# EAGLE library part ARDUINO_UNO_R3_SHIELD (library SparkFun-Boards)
Arduino R3 Shield Footprint Shield form compatible with the Arduino Uno R3. SparkFun Products: MG2639 Cellular Shield MIDI Shield R3 Stackable Headers Kit
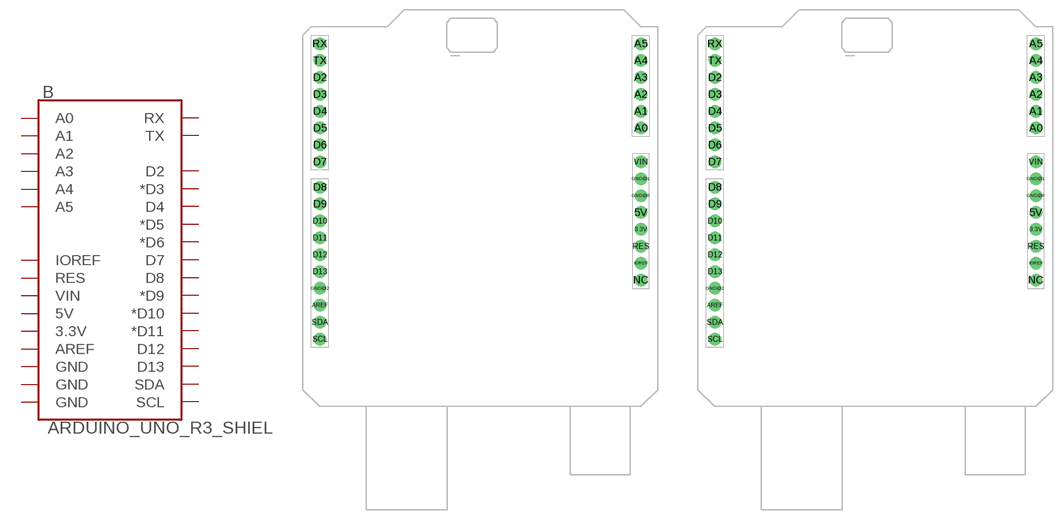
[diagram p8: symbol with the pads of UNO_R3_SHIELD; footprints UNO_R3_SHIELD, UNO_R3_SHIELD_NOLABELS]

Designator prefix B

## ARDUINO_UNO_R3_SHIELDBASIC  [UNO_R3_SHIELD]
3.3V  3.3V
5V  5V
A0  A0
A1  A1
A2  A2
A3  A3
A4  A4
A5  A5
AREF  AREF
D2  D2
D3  *D3
D4  D4
D5  *D5
D6  *D6
D7  D7
D8  D8
D9  *D9
D10  *D10
D11  *D11
D12  D12
D13  D13
GND@0  GND
GND@1  GND
GND@2  GND
IOREF  IOREF
RES  RES
RX  RX
SCL  SCL
SDA  SDA
TX  TX
VIN  VIN

## ARDUINO_UNO_R3_SHIELDNOLABELS  [UNO_R3_SHIELD_NOLABELS]
Pads as for UNO_R3_SHIELD

## ARDUINO_UNO_R3_SHIELDUNO_R3_SHIELD_LOCK  [UNO_R3_SHIELD_LOCK]
Pads as for UNO_R3_SHIELD

## ARDUINO_UNO_R3_SHIELDUNO_R3_SHIELD_NOLABELS_LOCK  [UNO_R3_SHIELD_NOLABELS_LOCK]
Pads as for UNO_R3_SHIELD

## Footprint UNO_R3_SHIELD (pad centres in mm)
Arduino Uno-Compatible Footprint No holes, no ICSP connections. Specifications: Pin count: 32 Pin pitch: 0.1" Area:2.1x2.35" Example device(s): Arduino Uno R3 Shield
drill 1.016 pad 1.88: 3.3V 24.13,-2.54; 5V 24.13,0; A0 24.13,12.7; A1 24.13,15.24; A2 24.13,17.78; A3 24.13,20.32; A4 24.13,22.86; A5 24.13,25.4; AREF -24.13,-13.97; D2 -24.13,20.32; D3 -24.13,17.78; D4 -24.13,15.24; D5 -24.13,12.7; D6 -24.13,10.16; D7 -24.13,7.62; D8 -24.13,3.81; D9 -24.13,1.27; D10 -24.13,-1.27; D11 -24.13,-3.81; D12 -24.13,-6.35; D13 -24.13,-8.89; GND@0 24.13,2.54; GND@1 24.13,5.08; GND@2 -24.13,-11.43; IOREF 24.13,-7.62; NC 24.13,-10.16; RES 24.13,-5.08; RX -24.13,25.4; SCL -24.13,-19.05; SDA -24.13,-16.51; TX -24.13,22.86; VIN 24.13,7.62

## Footprint UNO_R3_SHIELD_NOLABELS (pad centres in mm)
Arduino Uno-Compatible Footprint No holes, no ICSP connections, no silk labels. Specifications: Pin count: 32 Pin pitch: 0.1" Area:2.1x2.35" Example device(s): Arduino Uno R3 Shield
drill 1.016 pad 1.88: 3.3V 24.13,-3.81; 5V 24.13,-1.27; A0 24.13,11.43; A1 24.13,13.97; A2 24.13,16.51; A3 24.13,19.05; A4 24.13,21.59; A5 24.13,24.13; AREF -24.13,-15.24; D2 -24.13,19.05; D3 -24.13,16.51; D4 -24.13,13.97; D5 -24.13,11.43; D6 -24.13,8.89; D7 -24.13,6.35; D8 -24.13,2.54; D9 -24.13,0; D10 -24.13,-2.54; D11 -24.13,-5.08; D12 -24.13,-7.62; D13 -24.13,-10.16; GND@0 24.13,1.27; GND@1 24.13,3.81; GND@2 -24.13,-12.7; IOREF 24.13,-8.89; NC 24.13,-11.43; RES 24.13,-6.35; RX -24.13,24.13; SCL -24.13,-20.32; SDA -24.13,-17.78; TX -24.13,21.59; VIN 24.13,6.35

## Footprint UNO_R3_SHIELD_LOCK (pad centres in mm)
Arduino Uno-Compatible Footprint No holes, no ICSP connections. Locking footprint for headers. Specifications: Pin count: 32 Pin pitch: 0.1" Area:2.1x2.35" Example device(s): Arduino Uno R3 Shield
drill 1.016 pad 1.88: 3.3V 24.13,-3.81; 5V 24.384,-1.27; A0 24.384,11.43; A1 24.13,13.97; A2 24.384,16.51; A3 24.13,19.05; A4 24.384,21.59; A5 24.13,24.13; AREF -24.384,-15.24; D2 -24.13,19.05; D3 -24.384,16.51; D4 -24.13,13.97; D5 -24.384,11.43; D6 -24.13,8.89; D7 -24.384,6.35; D8 -24.13,2.54; D9 -24.384,0; D10 -24.13,-2.54; D11 -24.384,-5.08; D12 -24.13,-7.62; D13 -24.384,-10.16; GND@0 24.13,1.27; GND@1 24.384,3.81; GND@2 -24.13,-12.7; IOREF 24.13,-8.89; NC 24.384,-11.43; RES 24.384,-6.35; RX -24.13,24.13; SCL -24.13,-20.32; SDA -24.13,-17.78; TX -24.384,21.59; VIN 24.13,6.35

## Footprint UNO_R3_SHIELD_NOLABELS_LOCK (pad centres in mm)
Arduino Uno-Compatible Footprint No holes, no ICSP connections, no silk labels. Looking footprint for headers. Specifications: Pin count: 32 Pin pitch: 0.1" Area:2.1x2.35" Example device(s): Arduino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
drill 1.016 pad 1.88: 3.3V 24.13,-3.81; 5V 24.384,-1.27; A0 24.384,11.43; A1 24.13,13.97; A2 24.384,16.51; A3 24.13,19.05; A4 24.384,21.59; A5 24.13,24.13; AREF -24.384,-15.24; D2 -24.13,19.05; D3 -24.384,16.51; D4 -24.13,13.97; D5 -24.384,11.43; D6 -24.13,8.89; D7 -24.384,6.35; D8 -24.13,2.54; D9 -24.384,0; D10 -24.13,-2.54; D11 -24.384,-5.08; D12 -24.13,-7.62; D13 -24.384,-10.16; GND@0 24.13,1.27; GND@1 24.384,3.81; GND@2 -24.13,-12.7; IOREF 24.13,-8.89; NC 24.384,-11.43; RES 24.384,-6.35; RX -24.13,24.13; SCL -24.13,-20.32; SDA -24.13,-17.78; TX -24.384,21.59; VIN 24.13,6.35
